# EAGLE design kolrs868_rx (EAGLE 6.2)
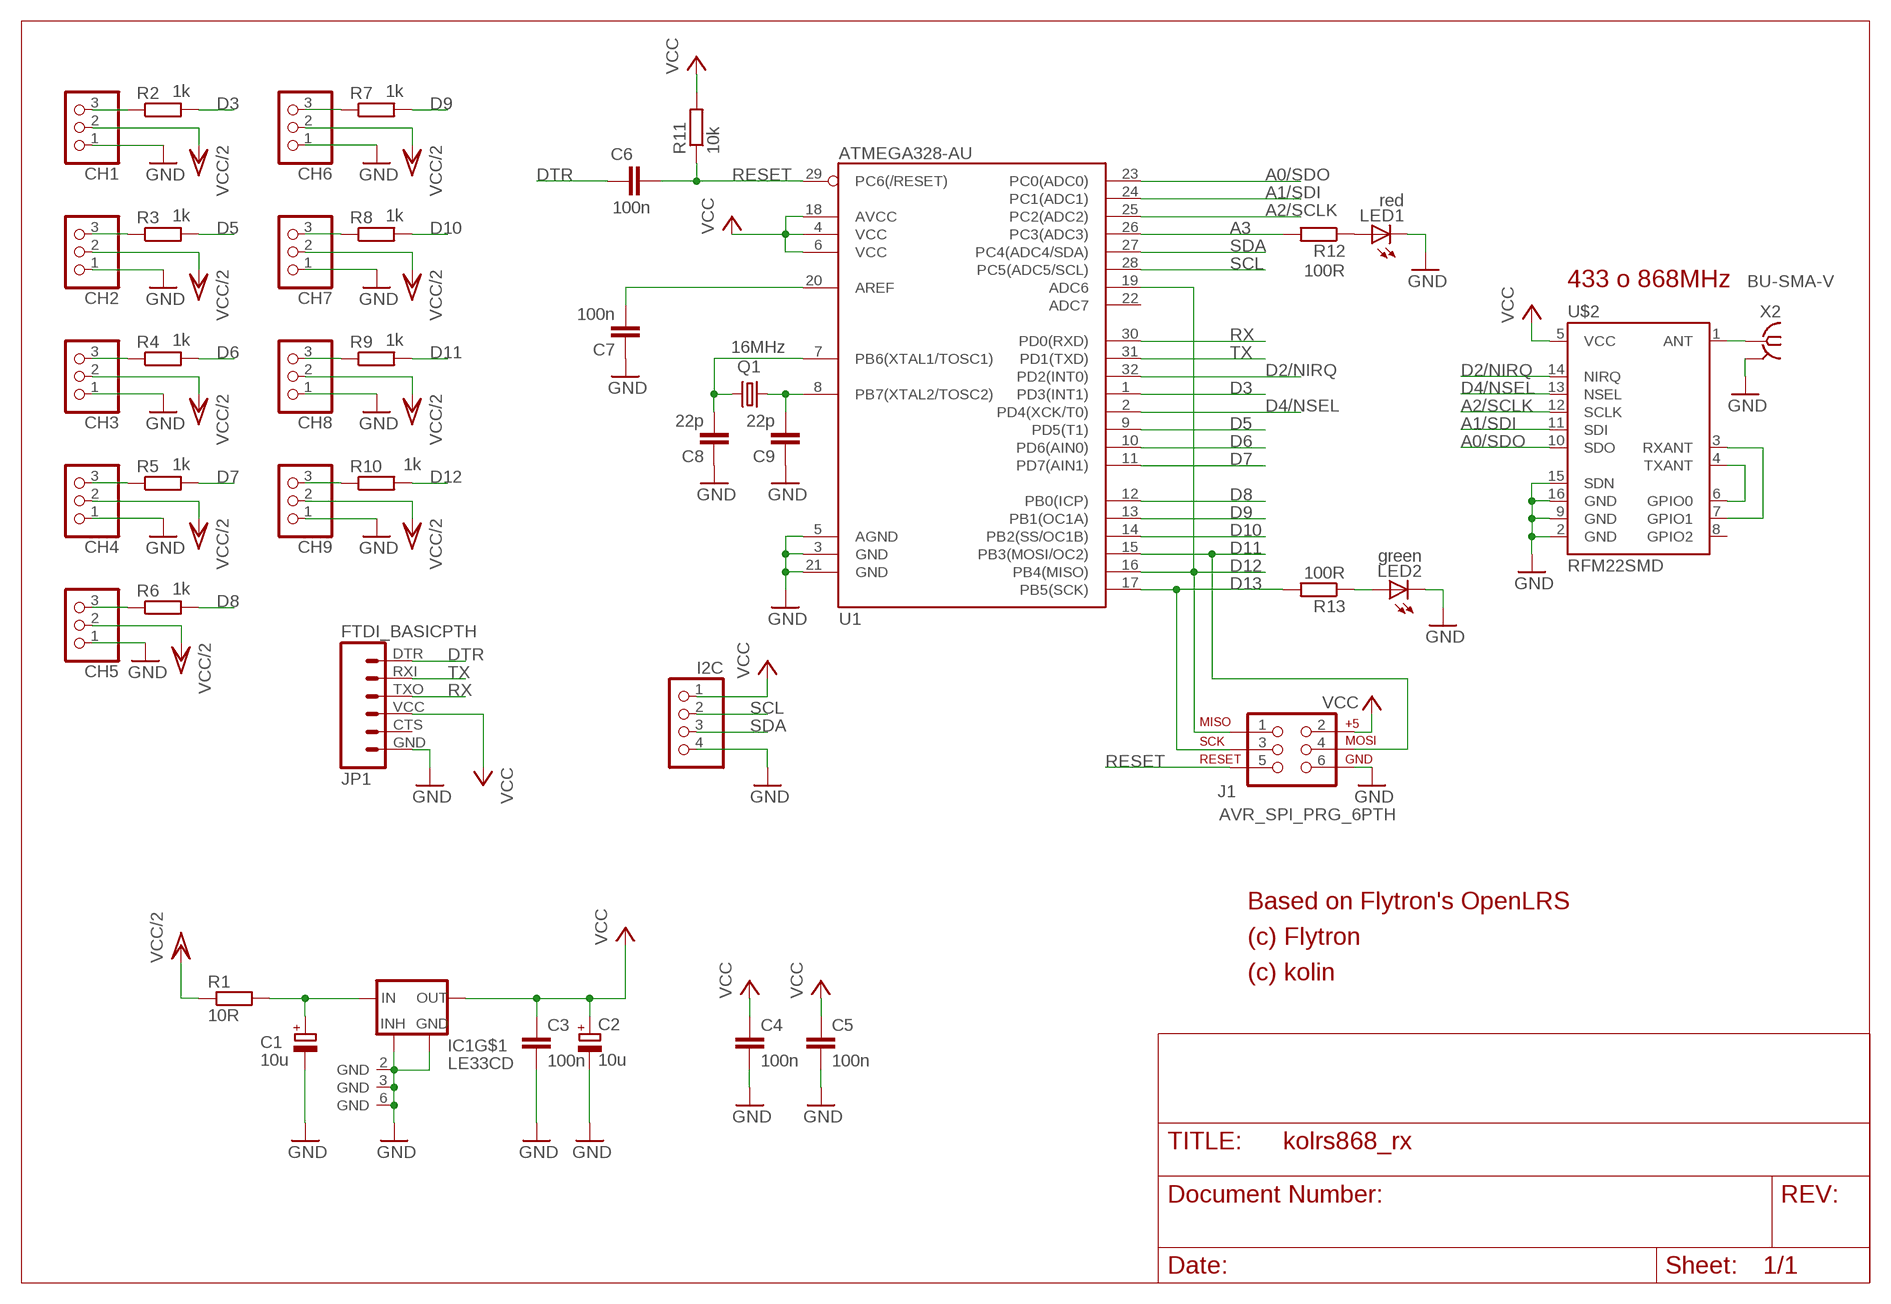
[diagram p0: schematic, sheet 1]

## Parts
C1  10u  CPOL-EUSMCB  [SMC_B]
C2  10u  CPOL-EUSMCB  [SMC_B]
C3  100n  C-EU_KOLIN  [M0805]
C4  100n  C-EU_KOLIN  [M0805]
C5  100n  C-EU_KOLIN  [M0805]
C6  100n  C-EU_KOLIN  [M0805]
C7  100n  C-EU_KOLIN  [M0805]
C8  22p  C-EU_KOLIN  [M0805]
C9  22p  C-EU_KOLIN  [M0805]
CH1  PINHD-1X3_KOLINOVO  [1X03]
CH2  PINHD-1X3_KOLINOVO  [1X03]
CH3  PINHD-1X3_KOLINOVO  [1X03]
CH4  PINHD-1X3_KOLINOVO  [1X03]
CH5  PINHD-1X3_KOLINOVO  [1X03]
CH6  PINHD-1X3_KOLINOVO  [1X03]
CH7  PINHD-1X3_KOLINOVO  [1X03]
CH8  PINHD-1X3_KOLINOVO  [1X03]
CH9  PINHD-1X3_KOLINOVO  [1X03]
I2C  PINHD-1X4  [1X04]
IC1  LE33CD  [SO8]
J1  AVR_SPI_PRG_6PTH  [2X3]
JP1  FTDI_BASICPTH  [FTDI_BASIC]
LED1  red  LEDCHIPLED_0805  [CHIPLED_0805]
LED2  green  LEDCHIPLED_0805  [CHIPLED_0805]
Q1  16MHz  CRYSTALHC49UP  [HC49UP]
R1  10R  R-EU_KOLINM0805  [M0805]
R2  1k  R-EU_KOLINM0805  [M0805]
R3  1k  R-EU_KOLINM0805  [M0805]
R4  1k  R-EU_KOLINM0805  [M0805]
R5  1k  R-EU_KOLINM0805  [M0805]
R6  1k  R-EU_KOLINM0805  [M0805]
R7  1k  R-EU_KOLINM0805  [M0805]
R8  1k  R-EU_KOLINM0805  [M0805]
R9  1k  R-EU_KOLINM0805  [M0805]
R10  1k  R-EU_KOLINM0805  [M0805]
R11  10k  R-EU_KOLINM0805  [M0805]
R12  100R  R-EU_KOLINM0805  [M0805]
R13  100R  R-EU_KOLINM0805  [M0805]
U1  ATMEGA328-AU  ATMEGA168  [TQFP32-08]
U$2  RFM22SMD  [RFM22-XXX-S2]
X2  BU-SMA-V  [BU-SMA-V]

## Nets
A0/SDO: U1.23(PC0(ADC0)) U$2.10(SDO)
A1/SDI: U1.24(PC1(ADC1)) U$2.11(SDI)
A2/SCLK: U1.25(PC2(ADC2)) U$2.12(SCLK)
A3: R12.2 U1.26(PC3(ADC3))
D2/NIRQ: U1.32(PD2(INT0)) U$2.14(NIRQ)
D3: R2.2 U1.1(PD3(INT1))
D4/NSEL: U1.2(PD4(XCK/T0)) U$2.13(NSEL)
D5: R3.2 U1.9(PD5(T1))
D6: R4.2 U1.10(PD6(AIN0))
D7: R5.2 U1.11(PD7(AIN1))
D8: R6.2 U1.12(PB0(ICP))
D9: R7.2 U1.13(PB1(OC1A))
D10: R8.2 U1.14(PB2(SS/OC1B))
D11: J1.4 R9.2 U1.15(PB3(MOSI/OC2))
D12: J1.1 R10.2 U1.16(PB4(MISO)) U1.19(ADC6)
D13: J1.3 R13.2 U1.17(PB5(SCK))
DTR: C6.1 JP1.DTR
GND: C1.- C2.- C3.2 C4.2 C5.2 C7.1 C8.1 C9.1 CH1.1 CH2.1 CH3.1 CH4.1 CH5.1 CH6.1 CH7.1 CH8.1 CH9.1 I2C.4 IC1.2(GND) IC1.3(GND) IC1.5(INHIBIT) IC1.6(GND) IC1.7(GND) J1.6 JP1.GND LED1.C LED2.C U1.3(GND) U1.5(AGND) U1.21(GND) U$2.2(GND) U$2.9(GND) U$2.15(SDN) U$2.16(GND) X2.2(GND)
N$1: C7.2 U1.20(AREF)
N$2: U$2.4(TXANT) U$2.6(GPIO0)
N$3: U$2.3(RXANT) U$2.7(GPIO1)
N$4: U$2.1(ANT) X2.1
N$5: LED1.A R12.1
N$6: C8.2 Q1.2 U1.7(PB6(XTAL1/TOSC1))
N$7: C9.2 Q1.1 U1.8(PB7(XTAL2/TOSC2))
N$9: C1.+ IC1.8(IN) R1.2
N$11: CH5.3 R6.1
N$12: CH1.3 R2.1
N$14: CH2.3 R3.1
N$15: CH3.3 R4.1
N$16: CH4.3 R5.1
N$17: CH6.3 R7.1
N$18: CH7.3 R8.1
N$19: CH8.3 R9.1
N$20: CH9.3 R10.1
N$25: LED2.A R13.1
RESET: C6.2 J1.5 R11.1 U1.29(PC6(/RESET))
RX: JP1.TXO U1.30(PD0(RXD))
SCL: I2C.2 U1.28(PC5(ADC5/SCL))
SDA: I2C.3 U1.27(PC4(ADC4/SDA))
TX: JP1.RXI U1.31(PD1(TXD))
VCC: C2.+ C3.1 C4.1 C5.1 I2C.1 IC1.1(OUT) J1.2 JP1.VCC R11.2 U1.4(VCC) U1.6(VCC) U1.18(AVCC) U$2.5(VCC)
VCC/2: CH1.2 CH2.2 CH3.2 CH4.2 CH5.2 CH6.2 CH7.2 CH8.2 CH9.2 R1.1
Unconnected: JP1.CTS U1.22(ADC7) U$2.8(GPIO2)

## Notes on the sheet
- 433 o 868MHz
- Based on Flytron's OpenLRS
- (c) Flytron
- (c) kolin

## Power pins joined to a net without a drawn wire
GND: X2.3(GND) X2.4(GND) X2.5(GND)

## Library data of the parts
C1 C2 = rcl:CPOL-EU: POLARIZED CAPACITOR, European symbol
C3-C9 = PINHEAD_RC:C-EU_KOLIN: CAPACITOR, European symbol
CH1-CH9 = PINHEAD_RC:PINHD-1X3_KOLINOVO: KOLINOVO PIN HEADER
I2C = pinhead:PINHD-1X4: PIN HEADER
IC1 = libstabilizatory:LE33CD: VOLTAGE REGULATOR WITH INHIBIT
J1 = SparkFun:AVR_SPI_PRG_6: AVR ISP 6 Pin This is the reduced ISP connector for AVR programming. Common on Arduino. This footprint will take up less PCB space and can be used with a 10-pin to 6-pin adapter such as SKU: BOB-08508
JP1 = SparkFun:FTDI_BASIC: FTDI Basic: 3.3V and 5V
LED1 LED2 = led:LED: LED
Q1 = crystal:CRYSTAL: CRYSTAL; OC_FARNELL: unknown; OC_NEWARK: unknown
R1-R13 = PINHEAD_RC:R-EU_KOLIN: RESISTOR, European symbol
U1 = SparkFun:ATMEGA168
U$2 = SparkFun:RFM22: Description: The RFM22 is a low-power, low cost radio that is capable of operating in the 434MHz and 900MHz open bands. It's frequency is software defined and there are some very good libraries written for it.
X2 = con-coax:BU-SMA-V: FEMALE SMA CONNECTOR Radiall distributor RS 112-3794; OC_FARNELL: unknown; OC_NEWARK: unknown

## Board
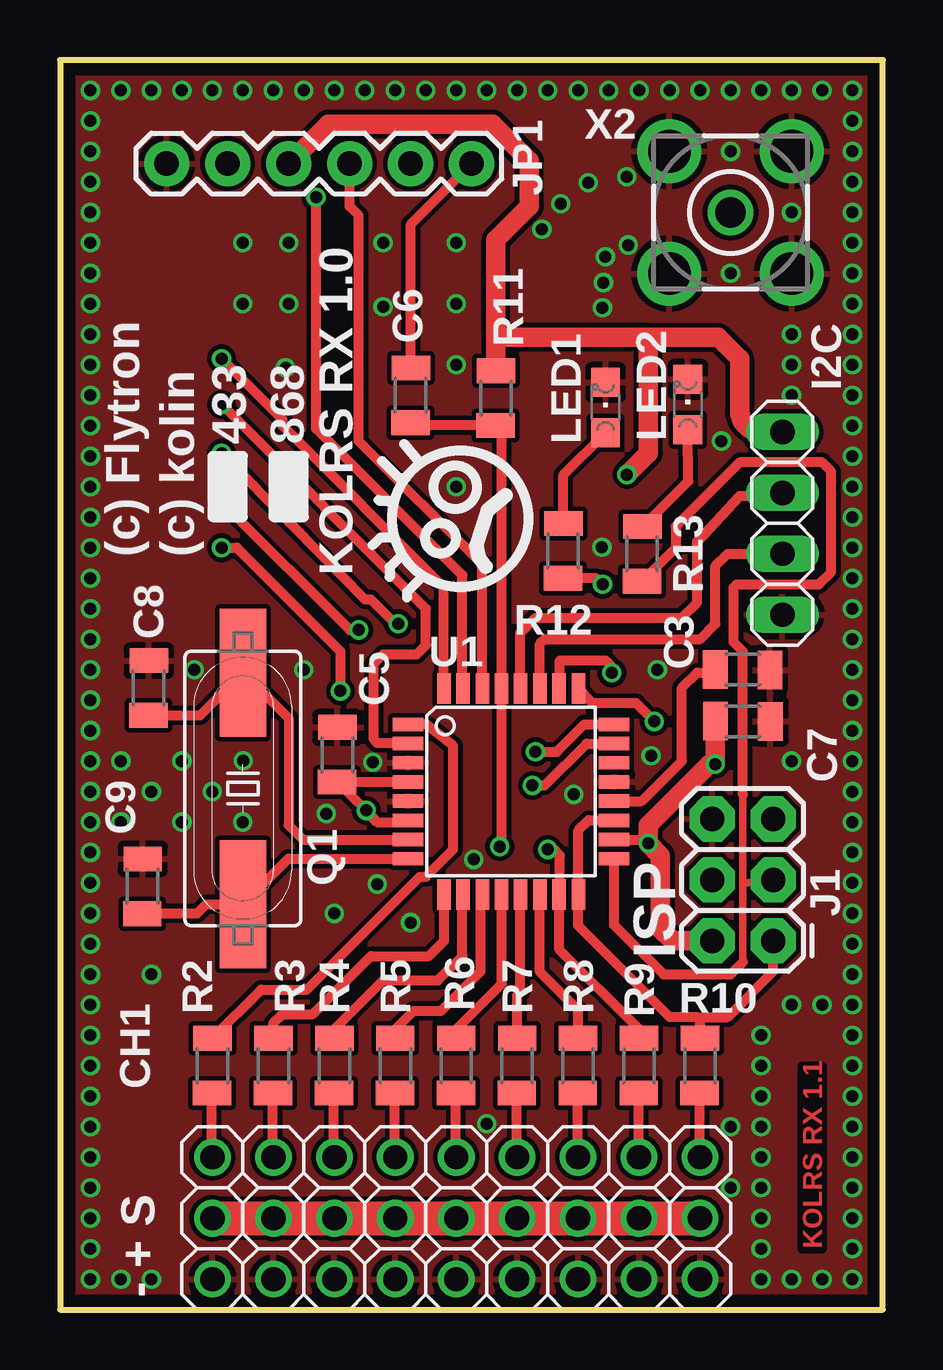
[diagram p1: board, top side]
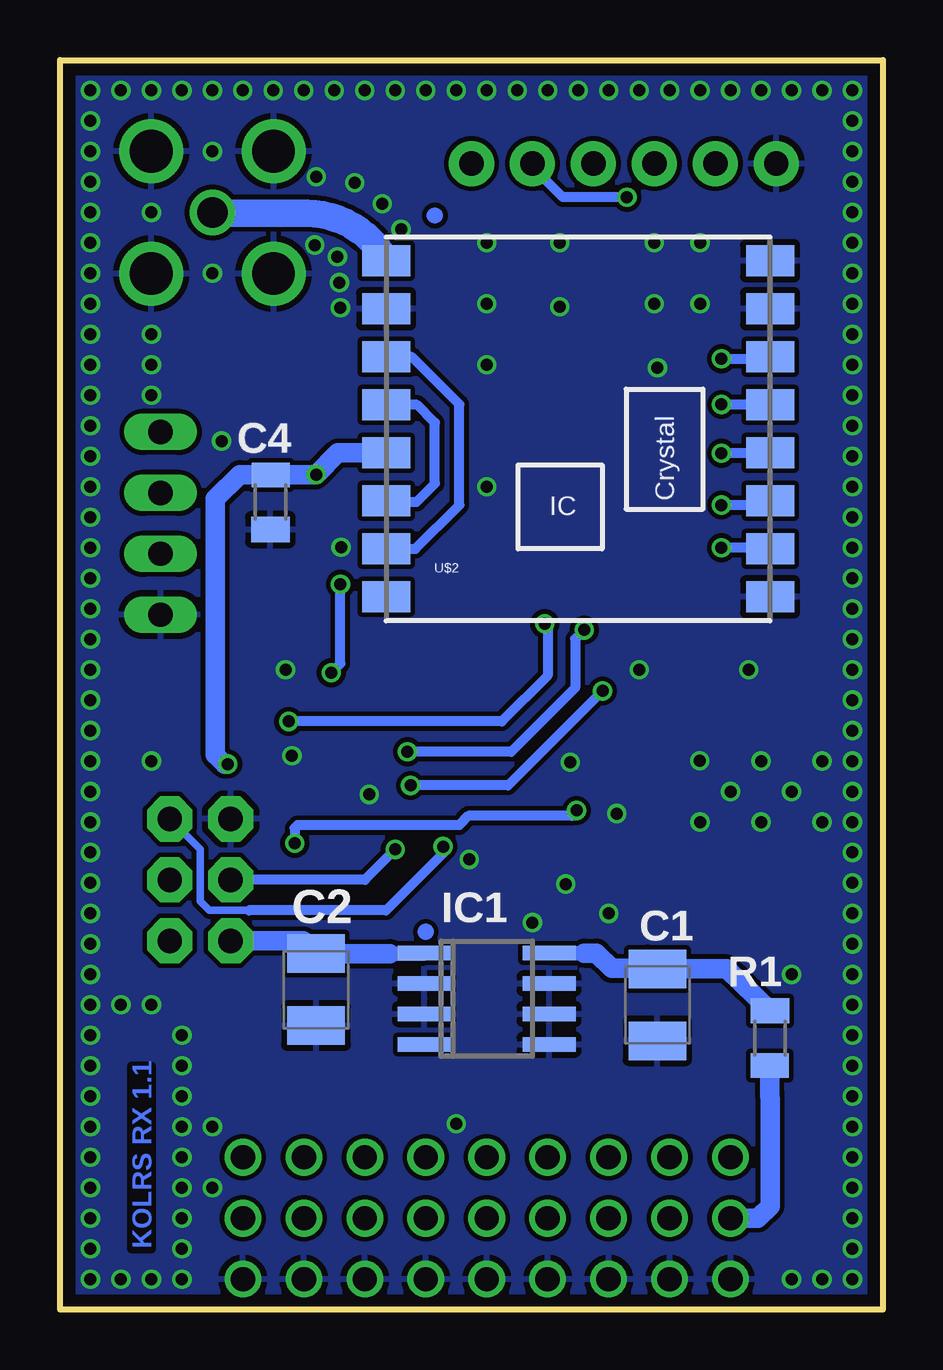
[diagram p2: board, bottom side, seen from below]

Size 34.29 x 52.07 mm. Coordinates in mm from the lower left corner, seen from the top.
Outline: 0,0 34.29,0 34.29,52.07 0,52.07 0,0
Copper layers (1*16): Top 0.018mm / dielectric 1.5mm / Bottom 0.018mm
Design rules: minimum track width 0.15mm, minimum drill 0.29mm, track to track 0.2mm, track to pad 0.2mm, pad to pad 0.2mm, via to via 0.2mm, smd to smd 0.2mm, copper to edge 20mil, drill to drill 8mil, minimum pad ring 0.15mm, minimum via ring 0.15mm, stop-mask expansion 4mil, vias tented up to drill 0.8mm, thermal gap 10mil

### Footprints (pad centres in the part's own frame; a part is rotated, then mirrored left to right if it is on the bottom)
SMC_B = smd 1.6 x 2.4: + -1.5,0; - 1.5,0
M0805 = smd 1.021 x 1.6: 1 -1.131,0.017 | smd 1.046 x 1.6: 2 1.148,0
1X03 = drill 1.016: 1 -2.54,0; 2 0,0; 3 2.54,0
1X04 = drill 1.016 long: 1 -3.81,0; 2 -1.27,0; 3 1.27,0; 4 3.81,0
SO8 = smd 0.6 x 2.2: 1 -1.905,-2.6; 2 -0.635,-2.6; 3 0.635,-2.6; 4 1.905,-2.6; 5 1.905,2.6; 6 0.635,2.6; 7 -0.635,2.6; 8 -1.905,2.6
2X3 = drill 1.016 pad 1.88 octagon: 1 0,0; 2 0,2.54; 3 2.54,0; 4 2.54,2.54; 5 5.08,0; 6 5.08,2.54
FTDI_BASIC = drill 1.016 pad 1.88: CTS 10.16,0; DTR 0,0; GND 12.7,0; RXI 2.54,0; TXO 5.08,0; VCC 7.62,0
CHIPLED_0805 = smd 1.2 x 1.2: A 0,-1.05; C 0,1.05
HC49UP = smd 5.334 x 1.93: 1 -4.826,0; 2 4.826,0
TQFP32-08 = smd 1.27 x 0.559: 1 -4.293,2.8; 2 -4.293,2; 3 -4.293,1.2; 4 -4.293,0.4; 5 -4.293,-0.4; 6 -4.293,-1.2; 7 -4.293,-2; 8 -4.293,-2.8; 17 4.293,-2.8; 18 4.293,-2; 19 4.293,-1.2; 20 4.293,-0.4; 21 4.293,0.4; 22 4.293,1.2; 23 4.293,2; 24 4.293,2.8 | smd 0.559 x 1.27: 9 -2.8,-4.293; 10 -2,-4.293; 11 -1.2,-4.293; 12 -0.4,-4.293; 13 0.4,-4.293; 14 1.2,-4.293; 15 2,-4.293; 16 2.8,-4.293; 25 2.8,4.293; 26 2,4.293; 27 1.2,4.293; 28 0.4,4.293; 29 -0.4,4.293; 30 -1.2,4.293; 31 -2,4.293; 32 -2.8,4.293
RFM22-XXX-S2 = smd 2 x 1.3: 1 -8,7; 2 -8,5; 3 -8,3; 4 -8,1; 5 -8,-1; 6 -8,-3; 7 -8,-5; 8 -8,-7; 9 8,-7; 10 8,-5; 11 8,-3; 12 8,-1; 13 8,1; 14 8,3; 15 8,5; 16 8,7
BU-SMA-V = drill 1.27: 1 0,0 | drill 1.778: 2 -2.55,2.55; 3 2.55,2.55; 4 2.55,-2.55; 5 -2.55,-2.55

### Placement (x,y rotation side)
C1  9.4,12.7 270 bottom
C2  23.62,13.34 270 bottom
C3  28.45,24.51 0 top
C4  25.53,33.65 270 bottom
C5  11.56,23.11 90 top
C6  14.61,38.1 270 top
C7  28.45,26.67 180 top
C8  3.68,25.91 270 top
C9  3.43,17.65 270 top
CH1  6.35,3.81 90 top
CH2  8.89,3.81 90 top
CH3  11.43,3.81 90 top
CH4  13.97,3.81 90 top
CH5  16.51,3.81 90 top
CH6  19.05,3.81 90 top
CH7  21.59,3.81 90 top
CH8  24.13,3.81 90 top
CH9  26.67,3.81 90 top
I2C  30.1,32.77 270 top
IC1  16.51,12.95 270 bottom
J1  29.72,15.37 90 top
JP1  17.14,47.75 180 top
LED1  22.73,37.59 0 top
LED2  26.16,37.72 0 top
Q1  7.62,21.72 90 top
R1  4.7,11.3 90 bottom
R2  6.35,10.16 90 top
R3  8.89,10.16 90 top
R4  11.43,10.16 90 top
R5  13.97,10.16 90 top
R6  16.51,10.16 90 top
R7  19.05,10.16 90 top
R8  21.59,10.16 90 top
R9  24.13,10.16 90 top
R10  26.67,10.16 90 top
R11  18.16,37.97 90 top
R12  20.96,31.62 270 top
R13  24.26,31.5 270 top
U1  18.8,21.59 0 top
U$2  12.7,36.7 0 bottom
X2  27.94,45.72 0 top

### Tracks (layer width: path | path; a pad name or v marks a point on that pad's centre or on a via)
A0/SDO  (via drill 0.5)
  Top 0.406: v6.73,31.75 7.37,31.75 11.68,27.43 v11.68,25.78 | U1.23 21.94,23.59 20.19,21.84 v19.68,21.84
  Bottom 0.406: U$2.10 4.75,31.75 v6.73,31.75 | v19.68,21.84 15.62,21.84 v11.68,25.78
A1/SDI  (via drill 0.5)
  Top 0.406: v6.73,33.53 6.86,33.53 12.07,28.32 v12.45,28.32 | U1.24 21.84,24.38 20.7,23.24 v19.81,23.24
  Bottom 0.406: U$2.11 4.88,33.53 v6.73,33.53 | v12.45,28.32 12.83,27.94 12.83,25.91 15.49,23.24 v19.81,23.24
A2/SCLK  (via drill 0.5)
  Top 0.406: U1.25 22.21,25.27 24,25.27 v24.77,24.51 | v6.73,35.69 12.7,29.59 12.95,29.59 13.97,28.57 v14.1,28.57
  Bottom 0.406: U$2.12 4.72,35.69 v6.73,35.69 | v14.1,28.57 13.97,28.45 13.97,26.42 15.88,24.51 v24.77,24.51
A3  (via drill 0.5)
  Top 0.406: U1.26 20.83,25.91 20.83,27.05 22.73,27.05 22.99,26.8 v22.99,26.54 | v22.61,30.23 22.36,30.48 R12.2
  Bottom 0.406: v22.99,26.54 22.61,26.92 v22.61,30.23
D2/NIRQ  (via drill 0.5)
  Top 0.406: U1.32 16,30.11 9.27,36.83 9.27,37.08 v6.73,39.62
  Bottom 0.406: U$2.14 4.78,39.62 v6.73,39.62
D3
  Top 0.406: R2.2 8.38,13.34 10.29,13.34 14.99,18.03 15.24,18.03 16.38,19.18 16.38,23.5 15.23,24.39 U1.1
D4/NSEL  (via drill 0.5)
  Top 0.406: U1.2 14.47,23.62 13.21,23.62 13.08,23.75 13.08,26.92 13.46,27.3 14.86,27.3 15.24,27.69 15.24,29.21 v6.73,37.72
  Bottom 0.406: v6.73,37.72 4.72,37.72 U$2.13
D5
  Top 0.406: U1.9 16,15.37 15.37,14.73 12.95,14.73 10.54,12.32 9.27,12.32 8.89,11.94 R3.2
D6
  Top 0.406: U1.10 16.76,17.27 16.76,14.73 15.75,13.72 13.46,13.72 11.43,11.68 R4.2
D7
  Top 0.406: U1.11 17.53,17.23 17.53,14.1 15.88,12.45 14.73,12.45 13.97,11.68 R5.2
D8
  Top 0.406: U1.12 18.41,17.28 18.41,13.59 16.51,11.68 R6.2
D9
  Top 0.406: U1.13 19.18,17.28 19.18,13.21 19.05,13.08 R7.2
D10
  Top 0.406: U1.14 20,14.07 21.59,12.48 R8.2
D11  (via drill 0.5)
  Top 0.406: R9.2 24.13,11.68 20.81,15 20.81,17.29 U1.15 20.83,17.33 20.83,18.92 20.57,19.18 v20.32,19.18
  Bottom 0.406: v20.32,19.18 21.59,17.91 J1.4
D12
  Top 0.406: U1.19 23.08,20.4 22.03,20.4 21.6,19.97 U1.16 21.6,16 25.4,12.19 26.54,12.19 26.67,12.07 | R10.2 26.67,12.07 | J1.1 29.72,14.1 27.81,12.19 26.8,12.19 26.67,12.07
D13
  Top 0.305: 28.45,21.46 28.45,18.47 28.45,17.78 | 28.45,14.48 28.45,17.78 | J1.3 29.59,17.78 28.45,17.78
  Top 0.406: 28.45,14.48 27.94,13.97 25.15,13.97 23.09,16.03 U1.17 | R13.2 25.65,31.75 25.65,32.64 28.32,35.31 31.75,35.31 32.13,34.92 32.13,30.73 31.62,30.23 28.19,30.23 28.07,30.1 28.07,27.81 28.45,27.43 28.45,21.46
DTR
  Top 0.406: JP1.DTR 14.62,45.23 C6.1
GND  (via drill 0.5)
  other vias: 21.41,21.47 1.27,1.27 1.27,3.81 3.81,1.27 1.27,6.35 1.27,8.89 1.27,11.43 1.27,13.97 1.27,16.51 1.27,19.05 1.27,21.59 3.81,21.59 6.35,21.59 11.43,16.51 1.27,24.13 1.27,26.67 1.27,29.21 1.27,31.75 1.27,34.29 1.27,36.83 1.27,41.91 1.27,44.45 1.27,46.99 1.27,49.53 2.54,50.8 7.62,50.8 10.16,50.8 12.7,50.8 15.24,50.8 17.78,50.8 20.32,50.8 22.86,50.8 25.4,50.8 27.94,50.8 30.48,50.8 33.02,50.8 10.16,26.67 22.01,46.95 27.94,43.18 30.48,45.72 27.94,48.26 33.02,48.26 33.02,45.72 33.02,43.18 33.02,40.64 30.48,40.64 33.02,38.1 30.48,38.1 33.02,35.56 33.02,33.02 33.02,30.48 33.02,27.94 33.02,25.4 30.48,22.86 33.02,20.32 33.02,17.78 33.02,15.24 33.02,12.7 33.02,10.16 27.94,7.62 33.02,7.62 33.02,5.08 27.94,5.08 33.02,2.54 31.75,1.27 29.21,1.27 3.81,13.97 11.09,20.67 13.22,17.73 24.63,23.08 22.58,31.77 16.51,34.29 16.51,39.37 16.51,41.91 16.51,44.45 7.62,44.45 7.62,41.91 5.08,50.8 1.27,39.37 13.46,41.78 13.46,44.45 9.53,41.91 9.53,44.45 9.4,39.24 5.59,26.67 14.61,16.13 24.89,26.67 1.27,22.86 1.27,20.32 1.27,17.78 1.27,15.24 1.27,12.7 1.27,10.16 1.27,7.62 1.27,5.08 1.27,2.54 2.54,1.27 1.27,25.4 1.27,27.94 1.27,30.48 1.27,33.02 1.27,35.56 1.27,38.1 1.27,40.64 1.27,43.18 1.27,45.72 1.27,48.26 1.27,50.8 3.81,50.8 6.35,50.8 8.89,50.8 11.43,50.8 13.97,50.8 16.51,50.8 19.05,50.8 21.59,50.8 24.13,50.8 26.67,50.8 29.21,50.8 31.75,50.8 33.02,49.53 33.02,46.99 33.02,44.45 33.02,41.91 33.02,39.37 33.02,36.83 33.02,34.29 33.02,31.75 33.02,29.21 33.02,26.67 33.02,21.59 33.02,19.05 33.02,16.51 33.02,13.97 33.02,11.43 33.02,8.89 33.02,6.35 33.02,3.81 30.48,1.27 7.62,20.32 5.08,20.32 2.54,20.32 2.54,22.86 5.08,22.86 13.03,22.81 23.62,47.2 20.86,46.09 20.08,45.02 22.6,41.74 22.65,42.8 22.73,43.87 23.68,44.36 17.24,18.76 7.63,22.88 33.02,24.13 33.02,22.86 17.78,7.75 31.75,12.7 30.48,12.7 29.21,11.43 29.21,10.16 29.21,8.89 29.21,7.62 29.21,6.35 29.21,5.08 29.21,3.81 29.21,2.54 33.02,1.27 27.56,36.2 30.48,39.37
  pour Bottom: -0.64,52.7 34.92,52.7 34.92,-0.64 -0.64,-0.64
  pour Top: -0.64,52.7 34.92,52.7 34.92,-0.64 -0.64,-0.64
N$1
  Top 0.406: C7.2 27.17,26.54 26.54,26.54 25.91,25.91 25.91,22.86 24.24,21.19 U1.20
N$2
  Bottom 0.406: U$2.4 19.41,37.7 18.67,36.96 18.67,34.42 19.43,33.65 20.65,33.65 U$2.6
N$3
  Bottom 0.406: U$2.3 19.64,39.7 17.65,37.72 17.65,33.53 19.48,31.7 U$2.7
N$4
  Bottom 1.143: U$2.1 arc-62 24.02,45.68 27.91,45.68
  Bottom 1.27: 27.91,45.68 arc90 X2.1
N$5
  Top 0.406: R12.1 20.97,34.78 LED1.A
N$6
  Top 0.406: C8.2 5.84,24.77 Q1.2 9.53,24.64 9.53,20.19 10.13,19.59 U1.7
N$7
  Top 0.406: C9.2 5.71,16.51 6.1,16.89 Q1.1 9.52,18.79 U1.8
N$9
  Bottom 0.61: IC1.8 12.45,14.86
  Bottom 0.813: R1.2 6.51,14.2 C1.+ | C1.+ 9.8,14.61 | 12.45,14.86 11.94,14.86 11.3,14.22 9.42,14.22 C1.+
N$11
  Top 0.406: CH5.3 16.49,6.37 R6.1
N$12
  Top 0.406: CH1.3 6.33,6.37 R2.1
N$14
  Top 0.406: CH2.3 8.87,6.37 R3.1
N$15
  Top 0.406: CH3.3 11.41,6.37 R4.1
N$16
  Top 0.406: CH4.3 13.95,6.37 R5.1
N$17
  Top 0.406: CH6.3 19.03,6.37 R7.1
N$18
  Top 0.406: CH7.3 21.57,6.37 R8.1
N$19
  Top 0.406: CH8.3 24.11,6.37 R9.1
N$20
  Top 0.406: CH9.3 26.65,6.37 R10.1
N$25
  Top 0.406: LED2.A 26.18,34.53 R13.1
RESET  (via drill 0.5)
  Top 0.406: C6.2 14.71,36.84 R11.1 18.4,36.59 U1.29 18.41,25.86 18.41,19.38 v18.33,19.3
  Bottom 0.305: 26.42,16.64 28.07,16.64 28.45,17.02 28.45,19.18 J1.5
  Bottom 0.406: 26.42,16.64 20.7,16.64 18.33,19.01 v18.33,19.3
RX
  Top 0.406: U1.30 17.59,25.89 17.59,31.06 12.45,36.2 12.45,45.59 12.07,45.97 JP1.TXO
SCL
  Top 0.406: U1.28 19.18,25.9 19.18,28.19 19.81,28.83 25.91,28.83 26.54,29.46 26.54,32 28.32,33.91 29.97,33.91 I2C.2
SDA
  Top 0.406: U1.27 20,27.74 20.19,27.94 26.67,27.94 27.3,28.57 27.3,30.99 27.81,31.5 I2C.3
TX  (via drill 0.5)
  Top 0.406: U1.31 16.76,25.91 16.76,30.61 10.67,36.7 v10.67,46.35
  Bottom 0.406: v10.67,46.35 13.34,46.35 14.61,47.62 JP1.RXI
VCC  (via drill 0.5)
  Top 0.406: U1.4 C5.1 v12.77,20.8 13.21,20.32 14.43,20.32 U1.6 | U1.18 23.12,19.56 24.38,19.56 v24.51,19.43
  Top 0.813: JP1.VCC 11.18,49.4 18.03,49.4 19.56,47.88 19.56,45.97 18.16,44.58 18.16,40.77 | 18.16,40.77 R11.2 | 28.32,37.46 28.32,39.62 27.43,40.51 24.51,40.51 | 28.32,37.46 28.32,37.34 | 24.51,40.51 18.41,40.51 18.16,40.77 | 24.51,40.51 24.51,35.69 v23.62,34.8 | J1.2 25.53,15.37 25.02,15.88 25.02,18.92 v24.51,19.43 24.51,20.19 27.05,22.73 v27.3,22.73 27.3,24.52 C3.1 | I2C.1 29.21,36.58 arc-90 28.32,37.46
  Bottom 0.406: v12.77,20.8 12.95,20.57 17.27,20.57 17.65,20.19 24.38,20.19 24.51,20.07 v24.51,19.43
  Bottom 0.61: 20.55,14.84 19.13,14.84 IC1.1
  Bottom 0.813: 20.55,14.84 C2.+ 24.15,15.37 J1.2 | 20.73,35.67 U$2.5 22.72,35.7 v23.62,34.8 23.63,34.79 C4.1 25.52,34.8 26.8,34.8 27.81,33.78 27.81,23.11 27.43,22.73 v27.3,22.73
VCC/2
  Top 1.422: CH1.2 CH2.2 CH3.2 CH4.2 CH5.2 CH6.2 CH7.2 CH8.2 CH9.2
  Bottom 0.813: CH1.2 5.21,3.81 4.7,4.32 4.7,8.64 4.71,9.03 R1.1
(copper drawn outside any net)
  shapes: Bottom circle x2

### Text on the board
Top: KOLRS RX 1.1
Bottom: KOLRS RX 1.1
tNames: 433 | 868 | (c) Flytron | (c) kolin | KOLRS RX 1.0 | ISP | - + S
